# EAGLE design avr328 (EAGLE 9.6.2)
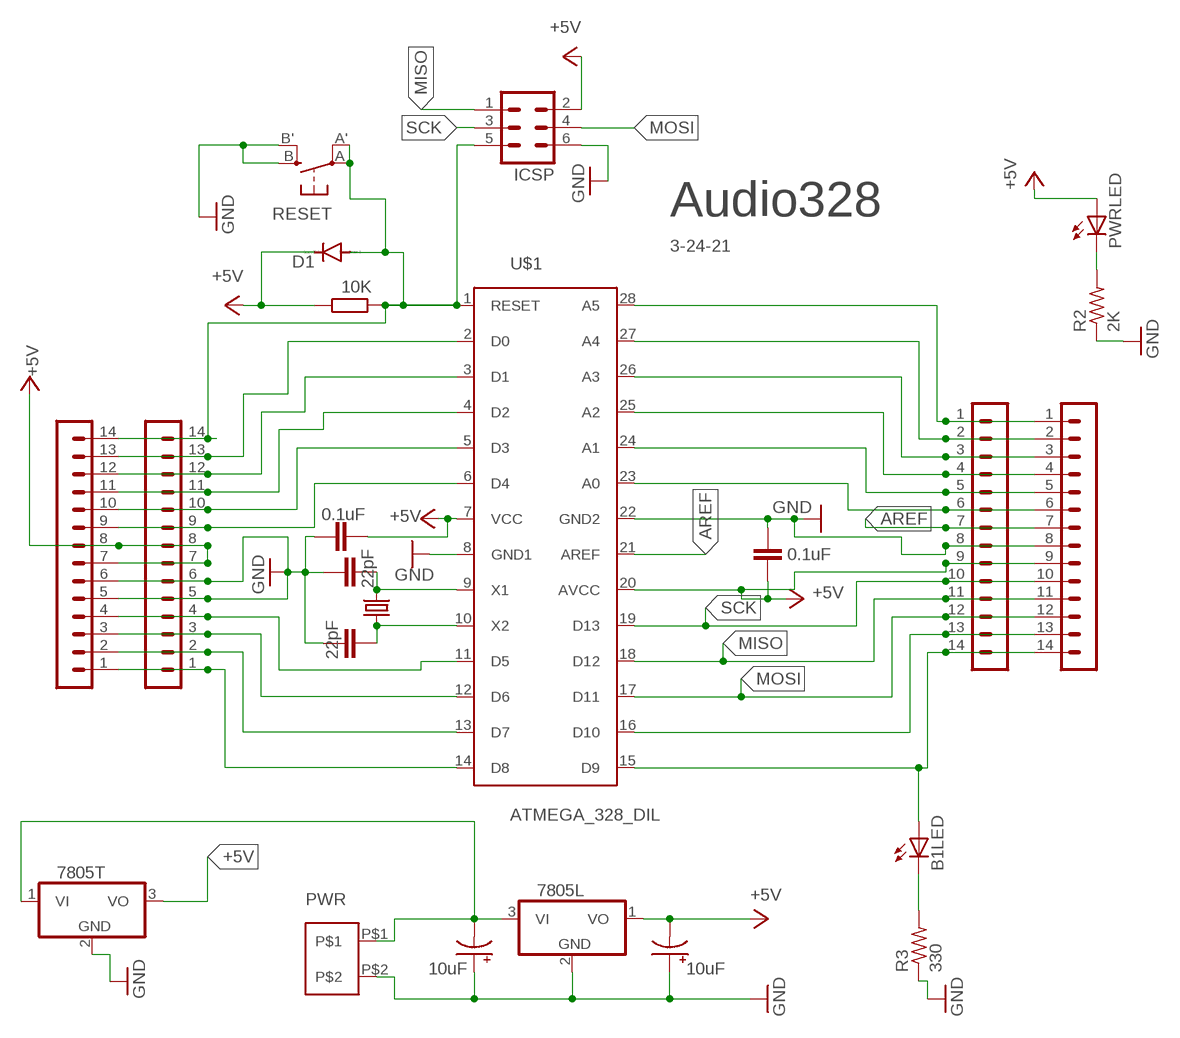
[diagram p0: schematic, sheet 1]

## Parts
-  14_PIN_CONN  [14_PIN_CONN]
.  14_PIN_CONN  [14_PIN_CONN]
.-  14_PIN_CONN  [14_PIN_CONN]
..  14_PIN_CONN  [14_PIN_CONN]
B1LED  LED3MM  [LED3MM]
C1  22pF  C-EU025-024X044  [C025-024X044]
C2  22pF  C-EU025-024X044  [C025-024X044]
C3  0.1uF  C-EU025-024X044  [C025-024X044]
C5  0.1uF  C-EU025-024X044  [C025-024X044]
C7  10uF  CPOL-USE2-5  [E2-5]
C8  10uF  CPOL-USE2-5  [E2-5]
D1  1N4148DO35-7  [DO35-7]
IC1  7805L  [TO92]
IC2  7805T  [TO220H]
ICSP  MA03-2  [MA03-2]
PWR  PWR  2_PIN_SCREW_CONN  [2_PIN_SCREW_CONN]
PWRLED  LED3MM  [LED3MM]
R1  10K  R-EU_0207/10  [0207/10]
R2  2K  R-US_0204/5  [0204/5]
R3  330  R-US_0204/5  [0204/5]
RESET  SPST_TACT-EVQQ2  [EVQ-Q2]
U$1  ATMEGA_328_DIL  [ATMEGA_328_DIL]
Y1  CRYSTALHC49UV  [HC49U-V]

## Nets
+5V [+5V]: -.9 .-.9 ..7 ..8 ...7 ...8 C3.2 C5.2 C7.- D1.C IC1.1(VO) IC2.3(VO) ICSP.2 PWRLED.A R1.1 U$1.7(VCC) U$1.20(AVCC)
AREF: -.7 .-.7 U$1.21(AREF)
GND: -.8 .-.8 ..5 ..6 ...5 ...6 C1.1 C2.1 C3.1 C5.1 C7.+ C8.+ IC1.2(GND) IC2.2(GND) ICSP.6 PWR.P$2 R2.1 R3.1 RESET.B'(S1) RESET.B(S) U$1.8(GND1) U$1.22(GND2)
MISO: -.11 .-.11 ICSP.1 U$1.18(D12)
MOSI: -.12 .-.12 ICSP.4 U$1.17(D11)
N$1: ..14 ...14 D1.A ICSP.5 R1.2 RESET.A'(P1) RESET.A(P) U$1.1(RESET)
N$2: C1.2 U$1.9(X1) Y1.2
N$3: C2.2 U$1.10(X2) Y1.1
N$4: ..13 ...13 U$1.2(D0)
N$5: ..12 ...12 U$1.3(D1)
N$6: ..11 ...11 U$1.4(D2)
N$7: C8.- IC1.3(VI) IC2.1(VI) PWR.P$1
N$8: ..9 ...9 U$1.6(D4)
N$10: -.1 .-.1 U$1.28(A5)
N$11: -.2 .-.2 U$1.27(A4)
N$12: -.3 .-.3 U$1.26(A3)
N$13: -.4 .-.4 U$1.25(A2)
N$14: -.5 .-.5 U$1.24(A1)
N$15: -.6 .-.6 U$1.23(A0)
N$16: -.14 .-.14 B1LED.A U$1.15(D9)
N$17: -.13 .-.13 U$1.16(D10)
N$18: B1LED.K(C) R3.2
N$19: PWRLED.K(C) R2.2
N$21: ..1 ...1 U$1.14(D8)
N$22: ..2 ...2 U$1.13(D7)
N$23: ..3 ...3 U$1.12(D6)
N$24: ..4 ...4 U$1.11(D5)
N$26: ..10 ...10 U$1.5(D3)
SCK: -.10 .-.10 ICSP.3 U$1.19(D13)

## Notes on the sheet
- Audio328
- 3-24-21

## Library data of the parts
- . .- .. = 14_PIN_CONN:14_PIN_CONN
B1LED PWRLED = adafruit:LED: LED
C1-C3 C5 = resistor:C-EU: CAPACITOR, European symbol
C7 C8 = rcl:CPOL-US: POLARIZED CAPACITOR, American symbol; SPICEPREFIX: C
D1 = diode:1N4148: DIODE
IC1 IC2 = adafruit:78*: Positive VOLTAGE REGULATOR Added bigger pads to the TO-92 package
ICSP = con-lstb:MA03-2: PIN HEADER; OC_FARNELL: unknown; OC_NEWARK: unknown
PWR = 2 Pin screw Conn:2_PIN_SCREW_CONN
R1 = resistor:R-EU_: RESISTOR, European symbol
R2 R3 = adafruit:R-US_: RESISTOR, American symbol
RESET = adafruit:SPST_TACT: SMT 6mm switch, EVQQ2 series http://www.ladyada.net/library/eagle
U$1 = Atmega_328_DIL:ATMEGA_328_DIL
Y1 = SparkFun-FreqCtrl:CRYSTAL: Various standard crystals. Proven footprints. Spark Fun Electronics SKU : COM-00534

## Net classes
1 +5V: width 0.381 mm

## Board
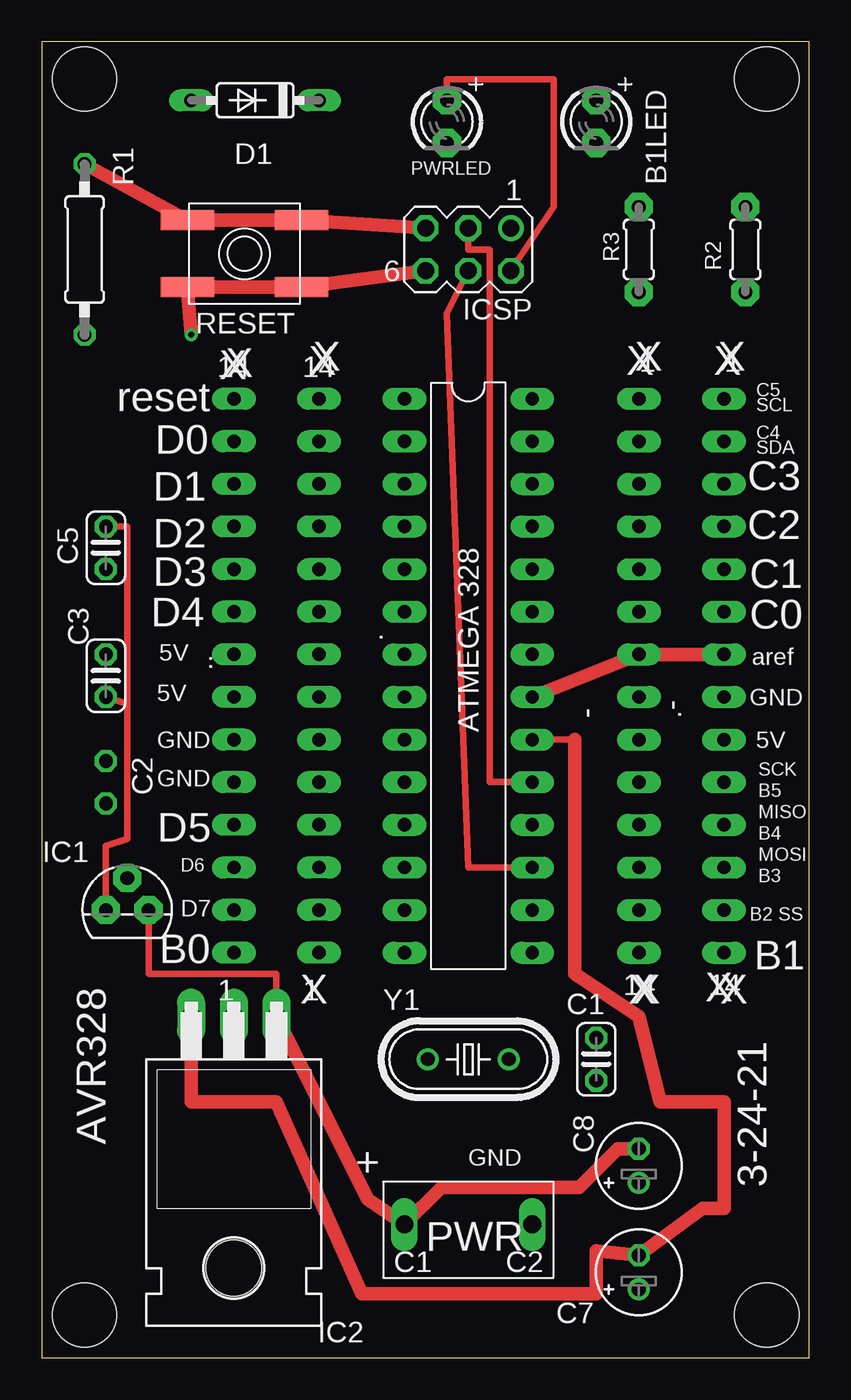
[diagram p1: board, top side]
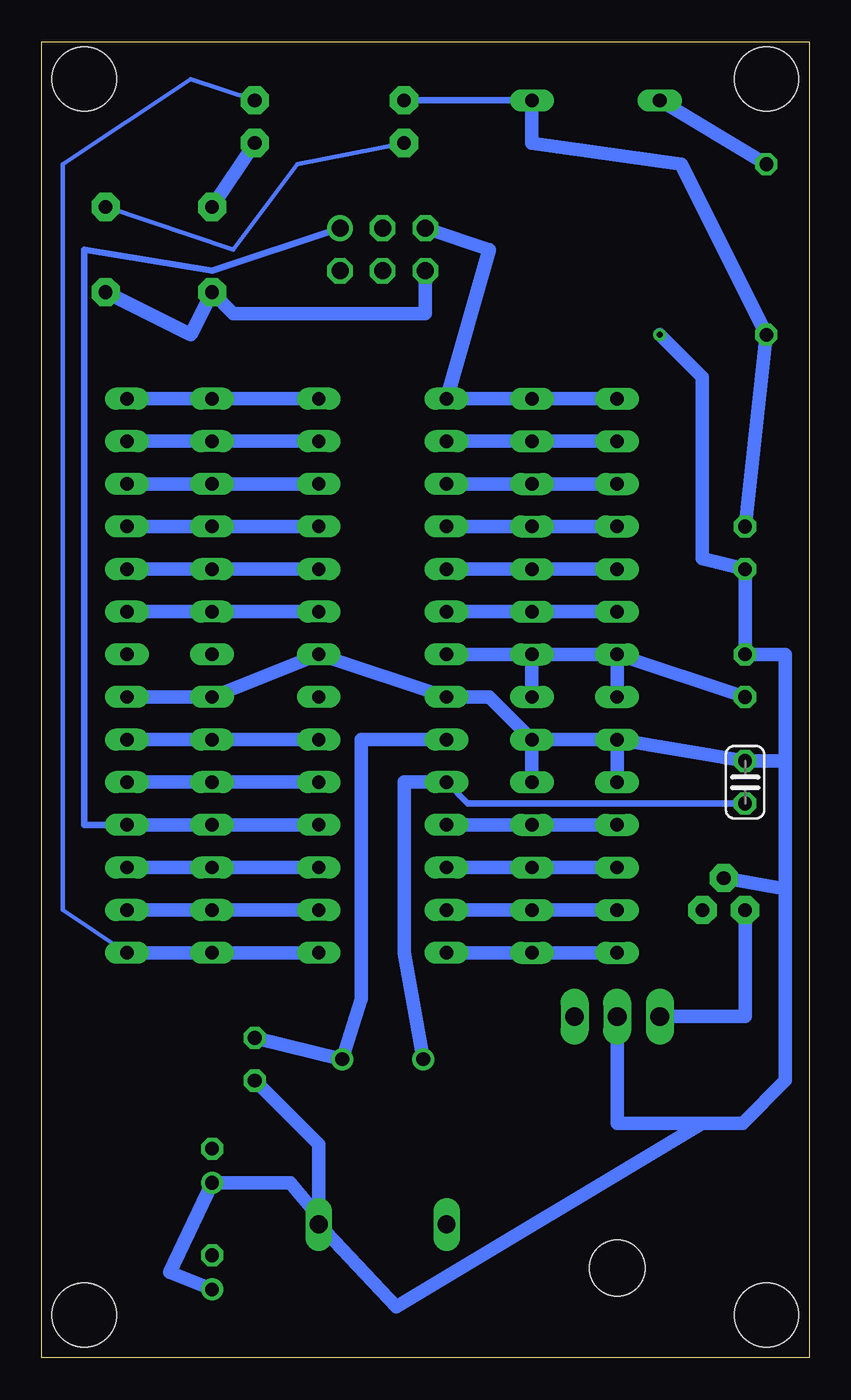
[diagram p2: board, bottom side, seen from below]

Size 45.7 x 78.41 mm. Coordinates in mm from the lower left corner, seen from the top.
Outline: 0,0 45.7,0 45.7,78.41 0,78.41 0,0
Copper layers (1*16): Top 0.035mm / dielectric 1.5mm / Bottom 0.035mm
Design rules "default": minimum track width 6mil, minimum drill 0.35mm, track to track 6mil, track to pad 6mil, pad to pad 6mil, via to via 6mil, smd to smd 6mil, copper to edge 40mil, drill to drill 6mil, minimum pad ring 10mil, minimum via ring 8mil, stop-mask expansion 4mil, vias tented up to drill 0mil, thermal gap 10mil
Holes 3.81 mm at 2.54,76.2 43.18,76.2 43.18,2.54 2.54,2.54

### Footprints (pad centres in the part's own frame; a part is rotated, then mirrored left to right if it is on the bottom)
14_PIN_CONN = drill 0.8 long: 1 -16.51,0; 2 -13.97,0; 3 -11.43,0; 4 -8.89,0; 5 -6.35,0; 6 -3.81,0; 7 -1.27,0; 8 1.27,0; 9 3.81,0; 10 6.35,0; 11 8.89,0; 12 11.43,0; 13 13.97,0; 14 16.51,0
LED3MM = drill 0.813 pad 1.676 octagon: A -1.27,0; K 1.27,0
C025-024X044 = drill 0.813 octagon: 1 -1.27,0; 2 1.27,0
E2-5 = drill 0.813 pad 1.27: + -1.016,0 | drill 0.813 pad 1.27 octagon: - 1.016,0
DO35-7 = drill 0.813 long: A 3.81,0; C -3.81,0
TO92 = drill 0.813 pad 1.676 octagon: 1 -1.27,0; 2 0,1.905; 3 1.27,0
TO220H = drill 1.118 long: 1 -2.54,-10.16; 2 0,-10.16; 3 2.54,-10.16 | hole 3.302: 0,4.826
MA03-2 = drill 1.016: 1 -2.54,-1.27 | drill 1.016 octagon: 2 -2.54,1.27; 3 0,-1.27; 4 0,1.27; 5 2.54,-1.27; 6 2.54,1.27
2_PIN_SCREW_CONN = drill 1.05 long: P$1 -3.81,0.318; P$2 3.81,0.318
0207/10 = drill 0.813 octagon: 1 -5.08,0; 2 5.08,0
0204/5 = drill 0.813 pad 1.676 octagon: 1 -2.54,0; 2 2.54,0
EVQ-Q2 = smd 3.2 x 1.2: A -3.4,-2; A' 3.4,-2; B -3.4,2; B' 3.4,2
ATMEGA_328_DIL = drill 0.8 long: 1 -16.51,-3.81; 2 -13.97,-3.81; 3 -11.43,-3.81; 4 -8.89,-3.81; 5 -6.35,-3.81; 6 -3.81,-3.81; 7 -1.27,-3.81; 8 1.27,-3.81; 9 3.81,-3.81; 10 6.35,-3.81; 11 8.89,-3.81; 12 11.43,-3.81; 13 13.97,-3.81; 14 16.51,-3.81; 15 16.51,3.81; 16 13.97,3.81; 17 11.43,3.81; 18 8.89,3.81; 19 6.35,3.81; 20 3.81,3.81; 21 1.27,3.81; 22 -1.27,3.81; 23 -3.81,3.81; 24 -6.35,3.81; 25 -8.89,3.81; 26 -11.43,3.81; 27 -13.97,3.81; 28 -16.51,3.81
HC49U-V = drill 0.813: 1 -2.413,0; 2 2.413,0

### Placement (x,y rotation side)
-  35.56,40.64 270 top
.  16.51,40.64 90 top
.-  40.64,40.64 270 top
..  11.43,40.64 90 top
B1LED  33.02,73.66 270 top
C1  33.02,17.78 90 top
C2  3.81,34.29 270 bottom
C3  3.81,40.64 270 top
C5  3.81,48.26 90 top
C7  35.56,5.08 90 top
C8  35.56,11.43 90 top
D1  12.7,74.93 180 top
IC1  5.08,26.67 0 top
IC2  11.43,10.16 180 top
ICSP  25.4,66.04 180 top
PWR  25.4,7.62 0 top
PWRLED  24.13,73.66 270 top
R1  2.54,66.04 90 top
R2  41.91,66.04 90 top
R3  35.56,66.04 90 top
RESET  12.06,65.79 180 top
U$1  25.4,40.64 270 top
Y1  25.4,17.78 0 top

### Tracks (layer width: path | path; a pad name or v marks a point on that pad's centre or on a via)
+5V
  Top 0.381: IC1.1 3.81,30.48 5.08,30.9 5.08,38.95 | 5.08,38.95 C3.2 | 5.08,38.95 5.08,49.53 C5.2 | ICSP.2 30.48,68.58 30.48,76.2 24.13,76.2 PWRLED.A | 31.75,36.83 U$1.20
  Top 0.813: IC2.3 8.89,15.24 13.97,15.24 19.05,3.81 33.02,3.81 33.02,6.35 C7.- 39.37,8.89 40.64,8.89 40.64,15.24 36.83,15.24 35.56,20.32 31.75,22.86 31.75,36.83
  Bottom 0.381: PWRLED.A D1.C
  Bottom 0.813: IC2.3 3.81,20.32 IC1.1 | ...8 ..8 | ..8 U$1.7 | C3.2 ...8 | D1.C 16.51,72.39 7.62,71.12 R1.1 C5.2 | ...7 ...8 | U$1.20 -.9 .-.9 | ..7 ..8
AREF
  Top 0.813: U$1.21 -.7 .-.7
GND  (via drill 0.35)
  Top 0.813: v8.89,60.96 RESET.B' RESET.B ICSP.6
  Bottom 0.813: PWR.P$2 29.21,8.38 30.9,10.41 C8.+ 38.1,5.08 C7.+ | C1.1 29.21,12.7 PWR.P$2 | PWR.P$2 24.59,3.03 6.35,13.97 | IC2.2 11.43,13.97 6.35,13.97 | 6.35,13.97 3.96,13.97 1.42,16.51 1.42,27.94 | 1.42,27.94 IC1.2 | 1.42,27.94 1.42,35.56 | 1.42,35.56 C2.1 ...6 | 1.42,35.56 1.42,41.91 C3.1 C5.1 6.35,47.62 6.35,58.42 v8.89,60.96 | ...6 ..6 | .-.8 -.8 U$1.22 U$1.8 19.05,39.37 ..6 | ..5 ..6 | ...5 ...6 | ICSP.6 22.86,62.23 34.29,62.23 R3.1 36.83,60.96 R2.1
MISO
  Bottom 0.381: ICSP.1 35.56,64.77 43.18,66.04 43.18,31.75 .-.11
  Bottom 0.813: U$1.18 -.11 .-.11
MOSI
  Top 0.381: U$1.17 25.4,29.21 24.13,62.23 ICSP.4
  Bottom 0.813: U$1.17 -.12 .-.12
N$1
  Top 0.813: ICSP.5 RESET.A RESET.A' R1.2
  Bottom 0.813: ICSP.5 19.05,66.04 U$1.1 ..14 ...14 | R1.2 D1.A
N$2
  Bottom 0.813: C1.2 Y1.2 26.67,21.39 26.67,36.83 U$1.9
N$3
  Bottom 0.381: C2.2 20.32,33.02 U$1.10
  Bottom 0.813: Y1.1 24.13,24.13 24.13,34.29 U$1.10
N$4
  Bottom 0.813: ...13 ..13 U$1.2
N$5
  Bottom 0.813: ...12 ..12 U$1.3
N$6
  Bottom 0.813: ...11 ..11 U$1.4
N$7
  Top 0.381: IC2.1 13.97,22.86 6.35,22.86 IC1.3
  Top 0.813: C8.- 34.29,12.45 32,10.16 23.81,10.16 PWR.P$1 19.41,9.43 IC2.1
N$8
  Bottom 0.813: ...9 ..9 U$1.6
N$10
  Bottom 0.813: U$1.28 -.1 .-.1
N$11
  Bottom 0.813: U$1.27 -.2 .-.2
N$12
  Bottom 0.813: U$1.26 -.3 .-.3
N$13
  Bottom 0.813: U$1.25 -.4 .-.4
N$14
  Bottom 0.813: U$1.24 -.5 .-.5
N$15
  Bottom 0.813: U$1.23 -.6 .-.6
N$16
  Bottom 0.254: .-.14 44.45,26.67 44.45,71.12 36.83,76.2 B1LED.A
  Bottom 0.813: U$1.15 -.14 .-.14
N$17
  Bottom 0.813: U$1.16 -.13 .-.13
N$18
  Bottom 0.813: R3.2 B1LED.K
N$19
  Bottom 0.254: R2.2 34.29,66.04 30.48,71.12 PWRLED.K
N$21
  Bottom 0.813: ...1 ..1 U$1.14
N$22
  Bottom 0.813: ...2 ..2 U$1.13
N$23
  Bottom 0.813: ...3 ..3 U$1.12
N$24
  Bottom 0.813: ...4 ..4 U$1.11
N$26
  Bottom 0.813: ...10 ..10 U$1.5
SCK
  Top 0.381: ICSP.3 25.4,66.04 26.67,66.04 26.67,34.29 U$1.19
  Bottom 0.813: U$1.19 -.10 .-.10

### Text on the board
tNames: X | X | X | X | X | X | X | X | C5 | reset | SCL | C4 | D0 | SDA | C3 | D1 | C2 | D2 | D3 | C1 | D4 | C0 | 5V | aref | 5V | GND | GND | 5V | SCK | GND | B5 | MISO | D5 | B4 | MOSI | D6 | B3 | D7 | B2 SS | B0 | B1 | X | X | X | X | X | AVR328 | + | GND | 3-24-21 | PWR

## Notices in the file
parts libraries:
SparkFun-FreqCtrl: Licensing: CC v3.0 Share-Alike You are welcome to use this library for commercial purposes.
